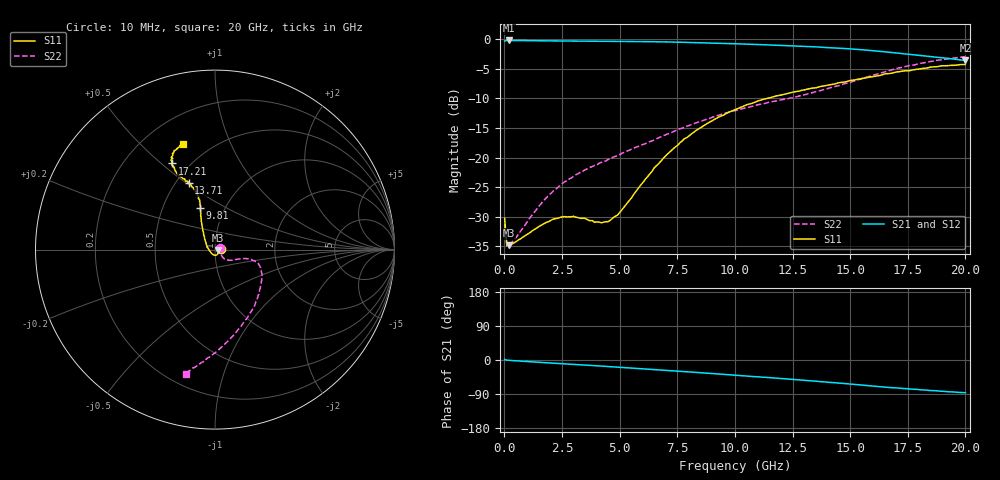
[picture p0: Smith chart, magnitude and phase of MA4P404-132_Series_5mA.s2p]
! AWR Design Environment (9226) Thu Aug 19 02:24:33 2021
! Document = '5mA'
! nPorts: 2, nXvals: 201
# GHz S DB R 50
!Freq DBS11 AngS11 DBS21 AngS21 DBS12 AngS12 DBS22 AngS22
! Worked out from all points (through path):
!   201 points, 10 MHz to 20 GHz, reference 50 ohm
!   highest |S21| = -0.21 dB at 210 MHz (marker M1); lowest = -3.6 dB at 20 GHz (marker M2)
!   group delay of S21, straight-line fit = 12.2 ps
!   lowest |S11| = -34.9 dB at 210 MHz (marker M3), VSWR 1.04, Z = 51.8 - j0.251 ohm
!   |S11| at or under -10 dB: start of sweep to 11.4 GHz
!   |S22| runs from -35.0 to -2.9 dB; largest |S21 - S12| = 0.033
!   S11 on the Smith chart (normalised r, x): 10 MHz: 1.06, +0.00; 9.81 GHz: 0.77, +0.38; 13.71 GHz: 0.58, +0.51; 17.21 GHz: 0.41, +0.55; 20 GHz: 0.36, +0.68
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0.01  -30.25 3.2  -0.29 1.2  -0.28 0.9  -31.33 16.2
0.11  -34.80 -5.9  -0.21 -0.4  -0.20 -0.4  -34.98 -6.8
0.21  -34.85 -7.7  -0.21 -0.9  -0.20 -0.9  -34.74 -8.4
1.61  -31.40 -51.0  -0.26 -6.5  -0.25 -6.2  -27.70 -39.2
2.11  -30.43 -64.5  -0.29 -8.3  -0.27 -8.0  -25.69 -43.3
2.61  -29.97 -78.1  -0.30 -10.2  -0.29 -9.8  -24.11 -44.9
3.41  -30.25 -100.8  -0.32 -13.1  -0.31 -12.6  -22.28 -43.6
4.21  -31.02 -136.6  -0.34 -16.1  -0.33 -15.5  -20.80 -39.3
4.51  -30.82 -151.1  -0.35 -17.3  -0.33 -16.6  -20.32 -37.9
4.91  -29.72 -174.3  -0.36 -18.8  -0.35 -18.1  -19.61 -34.5
6.71  -20.96 131.2  -0.44 -26.0  -0.42 -25.1  -16.65 -20.7
7.81  -16.82 119.4  -0.52 -30.6  -0.52 -29.5  -14.83 -16.1
9.81  -12.23 109.6  -0.74 -39.1  -0.73 -37.7  -12.26 -17.1
10.01  -11.90 108.4  -0.76 -40.1  -0.75 -38.5  -12.07 -17.3
11.71  -9.68 107.9  -1.00 -47.5  -0.94 -45.8  -10.50 -28.9
13.41  -8.25 111.0  -1.28 -55.3  -1.18 -53.7  -8.97 -47.8
13.71  -7.99 111.5  -1.34 -57.0  -1.24 -55.2  -8.69 -51.6
14.81  -7.20 114.4  -1.58 -62.4  -1.47 -60.7  -7.46 -65.2
16.71  -5.81 116.7  -2.21 -72.6  -2.09 -70.9  -5.28 -86.1
17.21  -5.43 116.3  -2.40 -74.8  -2.30 -73.5  -4.78 -90.1
18.71  -4.65 113.8  -3.03 -81.1  -3.01 -80.6  -3.60 -99.3
20  -4.25 106.9  -3.56 -86.6  -3.67 -85.7  -2.95 -103.2
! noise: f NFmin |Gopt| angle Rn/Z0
0.01  0  1  0  2e-20
2.21  0  1  0  2e-20
4.41  0  1  0  2e-20
6.61  0  1  0  2e-20
8.81  0  1  0  2e-20
11.11  0  1  0  2e-20
13.31  0  1  0  2e-20
15.51  0  1  0  2e-20
17.71  0  1  0  2e-20
20  0  1  0  2e-20
